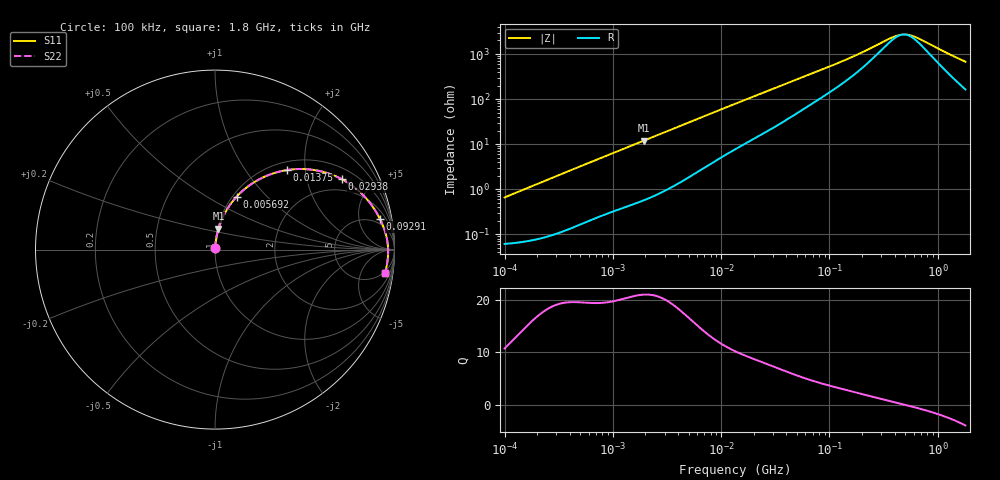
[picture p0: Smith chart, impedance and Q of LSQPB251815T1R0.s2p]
! LSQPB251815T1R0  S-PARAMETER MODEL  ( General Type )
! Model Generated by TAIYO YUDEN Corporation (http://www.ty-top.com)
! Version 3.0
! TAIYO YUDEN Control No. 130611NG22SB-FKC
! Copyright(c) 2010 TAIYO YUDEN CO.,LTD. All Rights Reserved.
! Product Description (link to TY-COMPAS)
! https://ds.yuden.co.jp/TYCOMPAS/or/detail?pn=LSQPB251815T1R0M&u=M
! Products Name : Inductors
! Characteristics :
!  Inductance : 1.0 uH , SRF(min) : 400 MHz , DC Resistance(max) : 0.0715 Ohm
!  Rated Current : Saturation :2000 mA , Temp Rise : 1400 mA (40 degC)
!  Case Size : 2.5 x 1.8 / 0.098 x 0.071 [mm/inch] , Thickness : 1.5 / 0.06 [mm/inch]
!  (Conditions: Temperature = 25 degC , DC Bias Current/Voltage = 0A / 0V)
! External Node Assignments :
!  1  o---GGG---o  2
! GND o---------o GND
! Frequency Range : 0.1MHz  -  1800MHz  [ 402 STEP ]
# MHz S RI R 50
! Freq[MHz].  S11 Real  S11 Imag  S21 Real  S21 Imag  S12 Real  S12 Imag  S22 Real  S22 Imag
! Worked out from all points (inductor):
!   401 points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, 100 kHz to 1.8 GHz, reference 50 ohm
!   read as one part in series: L = 1.04 uH near 105 kHz
!   highest Q = 21 at 1.937 MHz (marker M1), where L = 982 nH
!   self-resonance near 485.4 MHz
!   S11 on the Smith chart (normalised r, x): 100 kHz: 1.00, +0.01; 5.692 MHz: 1.04, +0.69; 13.75 MHz: 1.16, +1.59; 29.38 MHz: 1.44, +3.26; 92.91 MHz: 4, +9; 1.8 GHz: 4, -13
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0.1  0.00065 0.00652  0.9993 -0.00652  0.9993 -0.00652  0.00065 0.00652
0.516129  0.00278 0.0329  0.9972 -0.0329  0.9972 -0.0329  0.00278 0.0329
1.937403  0.0195 0.1165  0.9805 -0.1165  0.9805 -0.1165  0.0195 0.1165
2.66389  0.0333 0.1567  0.9667 -0.1567  0.9667 -0.1567  0.0333 0.1567
4.039851  0.0681 0.2261  0.9319 -0.2261  0.9319 -0.2261  0.0681 0.2261
5.692459  0.1208 0.2954  0.8792 -0.2954  0.8792 -0.2954  0.1208 0.2954
8.632747  0.2269 0.3808  0.7731 -0.3808  0.7731 -0.3808  0.2269 0.3808
13.41641  0.39 0.4412  0.61 -0.4412  0.61 -0.4412  0.39 0.4412
13.74911  0.4002 0.4429  0.5998 -0.4429  0.5998 -0.4429  0.4002 0.4429
19.85396  0.556 0.4429  0.444 -0.4429  0.444 -0.4429  0.556 0.4429
29.38042  0.7056 0.3931  0.2944 -0.3931  0.2944 -0.3931  0.7056 0.3931
44.5561  0.8193 0.3098  0.1807 -0.3098  0.1807 -0.3098  0.8193 0.3098
69.24595  0.8903 0.2218  0.1097 -0.2218  0.1097 -0.2218  0.8903 0.2218
92.90788  0.9185 0.172  0.0815 -0.172  0.0815 -0.172  0.9185 0.172
180.0045  0.9517 0.0864  0.0483 -0.0864  0.0483 -0.0864  0.9517 0.0864
357.3983  0.9631 0.0239  0.0369 -0.0239  0.0369 -0.0239  0.9631 0.0239
456.5984  0.9644 0.00473  0.0356 -0.00473  0.0356 -0.00473  0.9644 0.00473
503.6016  0.9646 -0.00285  0.0354 0.00285  0.0354 0.00285  0.9646 -0.00285
569.2172  0.9646 -0.0124  0.0354 0.0124  0.0354 0.0124  0.9646 -0.0124
675.6865  0.9643 -0.0261  0.0357 0.0261  0.0357 0.0261  0.9643 -0.0261
1216.359  0.9584 -0.0814  0.0416 0.0814  0.0416 0.0814  0.9584 -0.0814
1800  0.9472 -0.1313  0.0528 0.1313  0.0528 0.1313  0.9472 -0.1313
